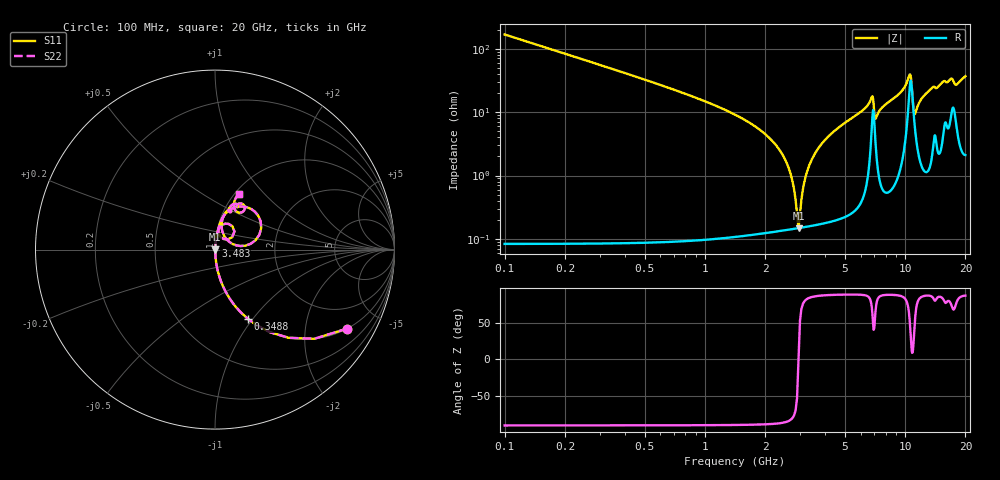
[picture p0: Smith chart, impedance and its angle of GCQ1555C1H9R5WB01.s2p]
!Murata Part Number: GCQ1555C1H9R5WB01
!These Parameters are Measured in Series Mode Connection
!Data Generated on Jan 08, 2026
!  o--ll--o
!Port1  Port2
!  o------o
!Operation Temp=25[degC], DC Bias Voltage=0[V]
!Freq. Start=100[MHz] Stop=20[GHz] 401[Steps]
# Hz S RI R 50
!Freq.(Hz) S11(Real) S11(Imag) S21(Real) S21(Imag) S12(Real) S12(Imag) S22(Real) S22(Imag)
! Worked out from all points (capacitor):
!   401 points, 100 MHz to 20 GHz, reference 50 ohm
!   read as one part in series: C = 9.5 pF near 199.5 MHz
!   lowest |Z| = 148 mohm at 2.936 GHz (marker M1)
!   series resonance near 2.935 GHz, so ESL is about 310 pH
!   S11 on the Smith chart (normalised r, x): 100 MHz: 1.00, -3.35; 348.8 MHz: 1.00, -0.95; 3.483 GHz: 1.00, +0.04; 20 GHz: 1.04, +0.74
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1e8  0.7368 -0.4401  0.2632 0.4401  0.2632 0.4401  0.7368 -0.4401
3.4875e8  0.1837 -0.3863  0.8163 0.3863  0.8163 0.3863  0.1837 -0.3863
9.955e8  0.0226 -0.1455  0.9774 0.1455  0.9774 0.1455  0.0226 -0.1455
2.33875e9  0.00201 -0.0262  0.998 0.0262  0.998 0.0262  0.00201 -0.0262
2.63725e9  0.00155 -0.0123  0.9984 0.0123  0.9984 0.0123  0.00155 -0.0123
2.93575e9  0.00148 1.29e-05  0.9985 -1.29e-05  0.9985 -1.29e-05  0.00148 1.29e-05
3.03525e9  0.00152 0.00386  0.9985 -0.00386  0.9985 -0.00386  0.00152 0.00386
3.1845e9  0.00163 0.00942  0.9984 -0.00942  0.9984 -0.00942  0.00163 0.00942
3.43325e9  0.00194 0.0182  0.9981 -0.0182  0.9981 -0.0182  0.00194 0.0182
3.483e9  0.00202 0.0199  0.998 -0.0199  0.998 -0.0199  0.00202 0.0199
4.3785e9  0.00425 0.0483  0.9957 -0.0483  0.9957 -0.0483  0.00425 0.0483
6.7665e9  0.058 0.1442  0.942 -0.1442  0.942 -0.1442  0.058 0.1442
7.1645e9  0.0289 0.0738  0.9711 -0.0738  0.9711 -0.0738  0.0289 0.0738
1.005e10  0.0941 0.2279  0.9059 -0.2279  0.9059 -0.2279  0.0941 0.2279
1.059725e10  0.2546 0.1564  0.7454 -0.1564  0.7454 -0.1564  0.2546 0.1564
1.0846e10  0.1692 0.0219  0.8308 -0.0219  0.8308 -0.0219  0.1692 0.0219
1.11445e10  0.0647 0.0575  0.9353 -0.0575  0.9353 -0.0575  0.0647 0.0575
1.199025e10  0.0376 0.148  0.9624 -0.148  0.9624 -0.148  0.0376 0.148
1.338325e10  0.0616 0.2102  0.9384 -0.2102  0.9384 -0.2102  0.0616 0.2102
1.67165e10  0.1385 0.2573  0.8615 -0.2573  0.8615 -0.2573  0.1385 0.2573
1.79105e10  0.1185 0.2136  0.8815 -0.2136  0.8815 -0.2136  0.1185 0.2136
2e10  0.1331 0.3124  0.8669 -0.3124  0.8669 -0.3124  0.1331 0.3124
